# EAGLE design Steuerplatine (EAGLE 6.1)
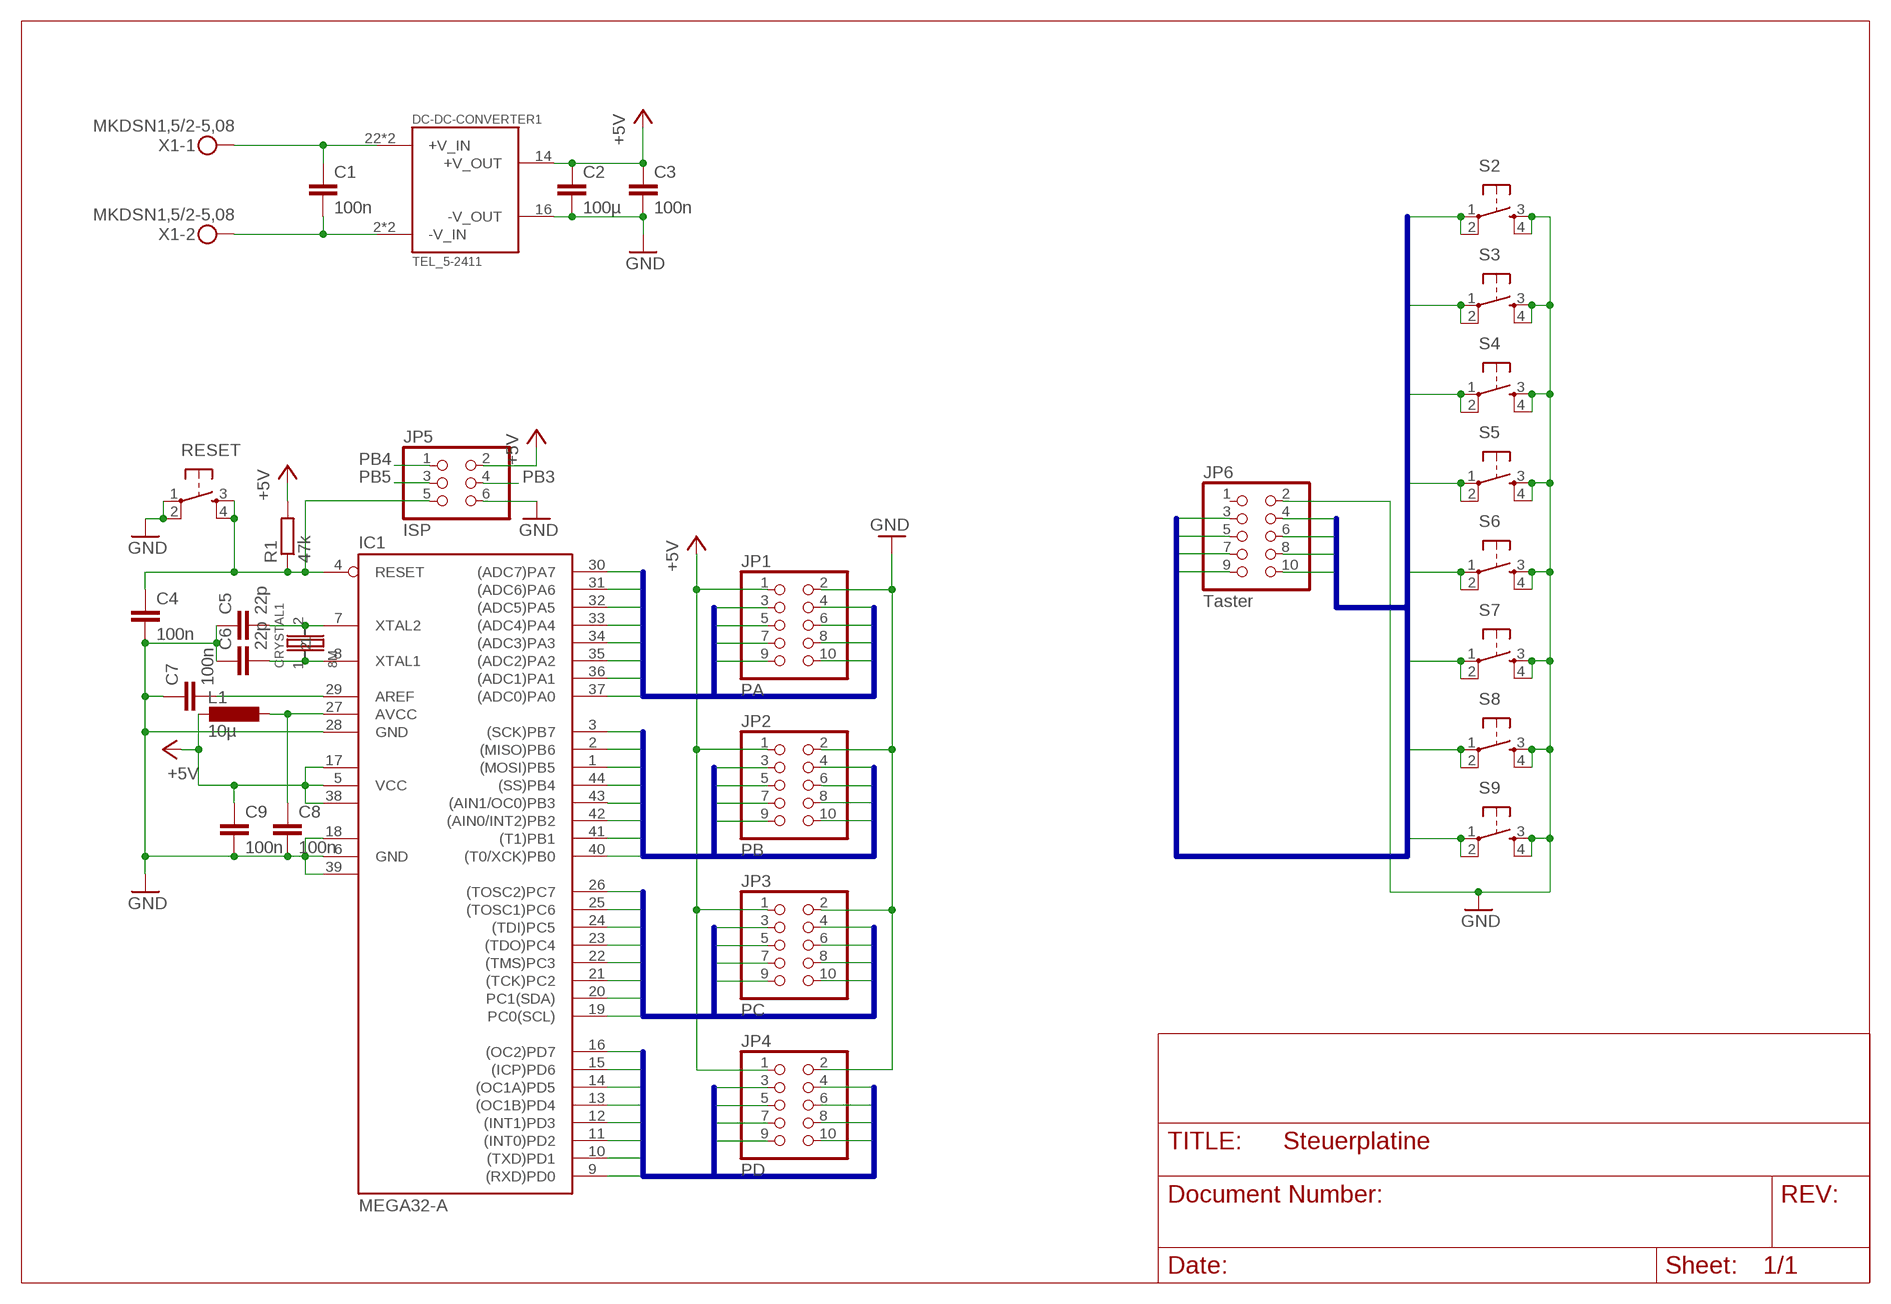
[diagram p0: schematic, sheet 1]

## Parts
C1  100n  C-EUC0603  [C0603]
C2  100µ  C-EUC1210  [C1210]
C3  100n  C-EUC0603  [C0603]
C4  100n  C-EUC0603  [C0603]
C5  22p  C-EUC0402  [C0402]
C6  22p  C-EUC0402  [C0402]
C7  100n  C-EUC0603  [C0603]
C8  100n  C-EUC0603  [C0603]
C9  100n  C-EUC0603  [C0603]
CRYSTAL1  8M  HC-49/SM  [HC-49/SM]
DC-DC-CONVERTER1  TEL_5-2411  [TEL_5-2411]
IC1  MEGA32-A  [TQFP44]
JP1  PA  PINHD-2X5  [2X05]
JP2  PB  PINHD-2X5  [2X05]
JP3  PC  PINHD-2X5  [2X05]
JP4  PD  PINHD-2X5  [2X05]
JP5  ISP  PINHD-2X3  [2X03]
JP6  Taster  PINHD-2X5  [2X05]
L1  10µ  L-EUL1812  [L1812]
R1  47k  R-EU_R0402  [R0402]
RESET  LSG  [SCHURTER_LSG]
S2  LSG  [SCHURTER_LSG]
S3  LSG  [SCHURTER_LSG]
S4  LSG  [SCHURTER_LSG]
S5  LSG  [SCHURTER_LSG]
S6  LSG  [SCHURTER_LSG]
S7  LSG  [SCHURTER_LSG]
S8  LSG  [SCHURTER_LSG]
S9  LSG  [SCHURTER_LSG]
X1  MKDSN1,5/2-5,08  [MKDSN1,5/2-5,08]

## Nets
+5V [5V]: C2.1 C3.1 C9.1 DC-DC-CONVERTER1.14(+V_OUT) IC1.5(VCC) IC1.17(VCC1) IC1.38(VCC2) JP1.1 JP2.1 JP3.1 JP4.1 JP5.2 L1.2 R1.2
GND [5V]: C2.2 C3.2 C4.2 C5.1 C6.1 C7.1 C8.2 C9.2 DC-DC-CONVERTER1.16(-V_OUT) IC1.6(GND) IC1.18(GND1) IC1.28(GND) IC1.39(GND2) JP1.2 JP2.2 JP3.2 JP4.2 JP5.6 JP6.2 RESET.1(P) RESET.2(P1) S2.3(S) S2.4(S1) S3.3(S) S3.4(S1) S4.3(S) S4.4(S1) S5.3(S) S5.4(S1) S6.3(S) S6.4(S1) S7.3(S) S7.4(S1) S8.3(S) S8.4(S1) S9.3(S) S9.4(S1)
N$1 [24V In]: C1.1 DC-DC-CONVERTER1.22(+V_IN) DC-DC-CONVERTER1.23(+V_IN) X1.1
N$2 [24V In]: C1.2 DC-DC-CONVERTER1.2(-V_IN) DC-DC-CONVERTER1.3(-V_IN) X1.2
N$3 [5V]: C4.1 IC1.4(RESET) JP5.5 R1.1 RESET.3(S) RESET.4(S1)
N$4 [5V]: C5.2 CRYSTAL1.2 IC1.7(XTAL2)
N$5 [5V]: C6.2 CRYSTAL1.1 IC1.8(XTAL1)
N$6 [5V]: C7.2 IC1.29(AREF)
N$7: C8.1 IC1.27(AVCC) L1.1
PA0 [5V]: IC1.37((ADC0)PA0) JP1.3
PA1 [5V]: IC1.36((ADC1)PA1) JP1.4
PA2 [5V]: IC1.35((ADC2)PA2) JP1.5
PA3 [5V]: IC1.34((ADC3)PA3) JP1.6
PA4 [5V]: IC1.33((ADC4)PA4) JP1.7
PA5 [5V]: IC1.32((ADC5)PA5) JP1.8
PA6 [5V]: IC1.31((ADC6)PA6) JP1.9
PA7 [5V]: IC1.30((ADC7)PA7) JP1.10
PB0 [5V]: IC1.40((T0/XCK)PB0) JP2.3
PB1 [5V]: IC1.41((T1)PB1) JP2.4
PB2 [5V]: IC1.42((AIN0/INT2)PB2) JP2.5
PB3: IC1.43((AIN1/OC0)PB3) JP2.6 JP5.4
PB4: IC1.44((SS)PB4) JP2.7 JP5.1
PB5 [5V]: IC1.1((MOSI)PB5) JP2.8 JP5.3
PB6 [5V]: IC1.2((MISO)PB6) JP2.9
PB7 [5V]: IC1.3((SCK)PB7) JP2.10
PC0 [5V]: IC1.19(PC0(SCL)) JP3.3
PC1 [5V]: IC1.20(PC1(SDA)) JP3.4
PC2 [5V]: IC1.21((TCK)PC2) JP3.5
PC3 [5V]: IC1.22((TMS)PC3) JP3.6
PC4 [5V]: IC1.23((TDO)PC4) JP3.7
PC5 [5V]: IC1.24((TDI)PC5) JP3.8
PC6 [5V]: IC1.25((TOSC1)PC6) JP3.9
PC7 [5V]: IC1.26((TOSC2)PC7) JP3.10
PD0 [5V]: IC1.9((RXD)PD0) JP4.3
PD1 [5V]: IC1.10((TXD)PD1) JP4.4
PD2 [5V]: IC1.11((INT0)PD2) JP4.5
PD3 [5V]: IC1.12((INT1)PD3) JP4.6
PD4 [5V]: IC1.13((OC1B)PD4) JP4.7
PD5 [5V]: IC1.14((OC1A)PD5) JP4.8
PD6 [5V]: IC1.15((ICP)PD6) JP4.9
PD7 [5V]: IC1.16((OC2)PD7) JP4.10
TASTER3 [5V]: JP6.3 S2.1(P) S2.2(P1)
TASTER4 [5V]: JP6.4 S3.1(P) S3.2(P1)
TASTER5 [5V]: JP6.5 S4.1(P) S4.2(P1)
TASTER6 [5V]: JP6.6 S5.1(P) S5.2(P1)
TASTER7 [5V]: JP6.7 S6.1(P) S6.2(P1)
TASTER8 [5V]: JP6.8 S7.1(P) S7.2(P1)
TASTER9 [5V]: JP6.9 S8.1(P) S8.2(P1)
TASTER10 [5V]: JP6.10 S9.1(P) S9.2(P1)
Unconnected: JP6.1

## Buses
PA[0..7]
PB[0..7]
PC[0..7]
PD[0..7]
TASTER[1..10]

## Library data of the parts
C1-C9 = rcl:C-EU: CAPACITOR, European symbol
CRYSTAL1 = Bachelorarbeit_lib_Jonas:HC-49/SM: Quarz
DC-DC-CONVERTER1 = Bachelorarbeit_lib_Jonas:TEL_5-2411: DCDC Wandler TRACOPOWER TEL 5-2411 Link http://de.farnell.com/tracopower/tel-5-2411/wandler-dc-dc-5w-5v/dp/1242622?Ntt=tel5+2411
IC1 = atmel:MEGA32: MICROCONTROLLER 32 Kbytes FLASH 2 Kbytes SRAM 1 Kbytes EEPROM USART 8-channel 10 bit ADC Source: www.atmel.com .. doc2503.pdf; MPN: ATMEGA32-16AU; OC_FARNELL: 9171274; OC_NEWARK: 69K6677
JP1-JP4 JP6 = pinhead:PINHD-2X5: PIN HEADER
JP5 = pinhead:PINHD-2X3: PIN HEADER
L1 = rcl:L-EU: INDUCTOR, European symbol
R1 = rcl:R-EU_: RESISTOR, European symbol
RESET S2-S9 = switch-omron-smd:LSG
X1 = con-phoenix-508:MKDSN1,5/2-5,08: MKDSN 1,5/ 2-5,08 Printklemme; MPN: MKDSN 1,5/2-5.08; OC_FARNELL: 1792903; OC_NEWARK: 30M2397

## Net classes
1 24V In: width 0.254 mm, drill 0.584 mm
2 5V: width 0.203 mm, drill 0.584 mm

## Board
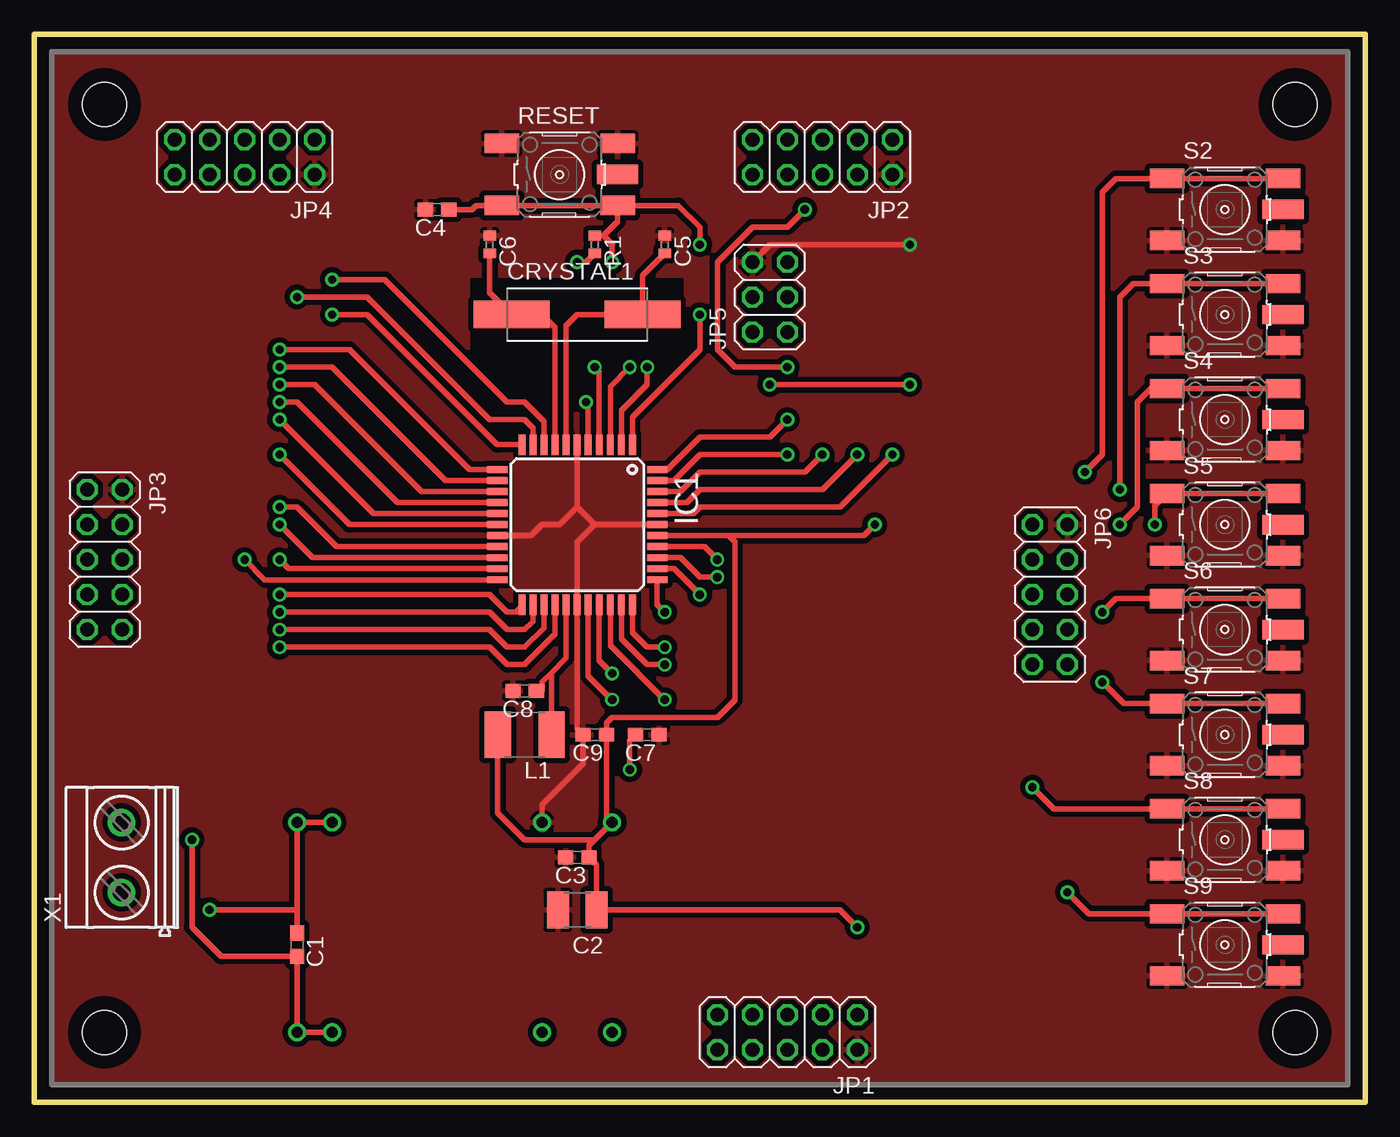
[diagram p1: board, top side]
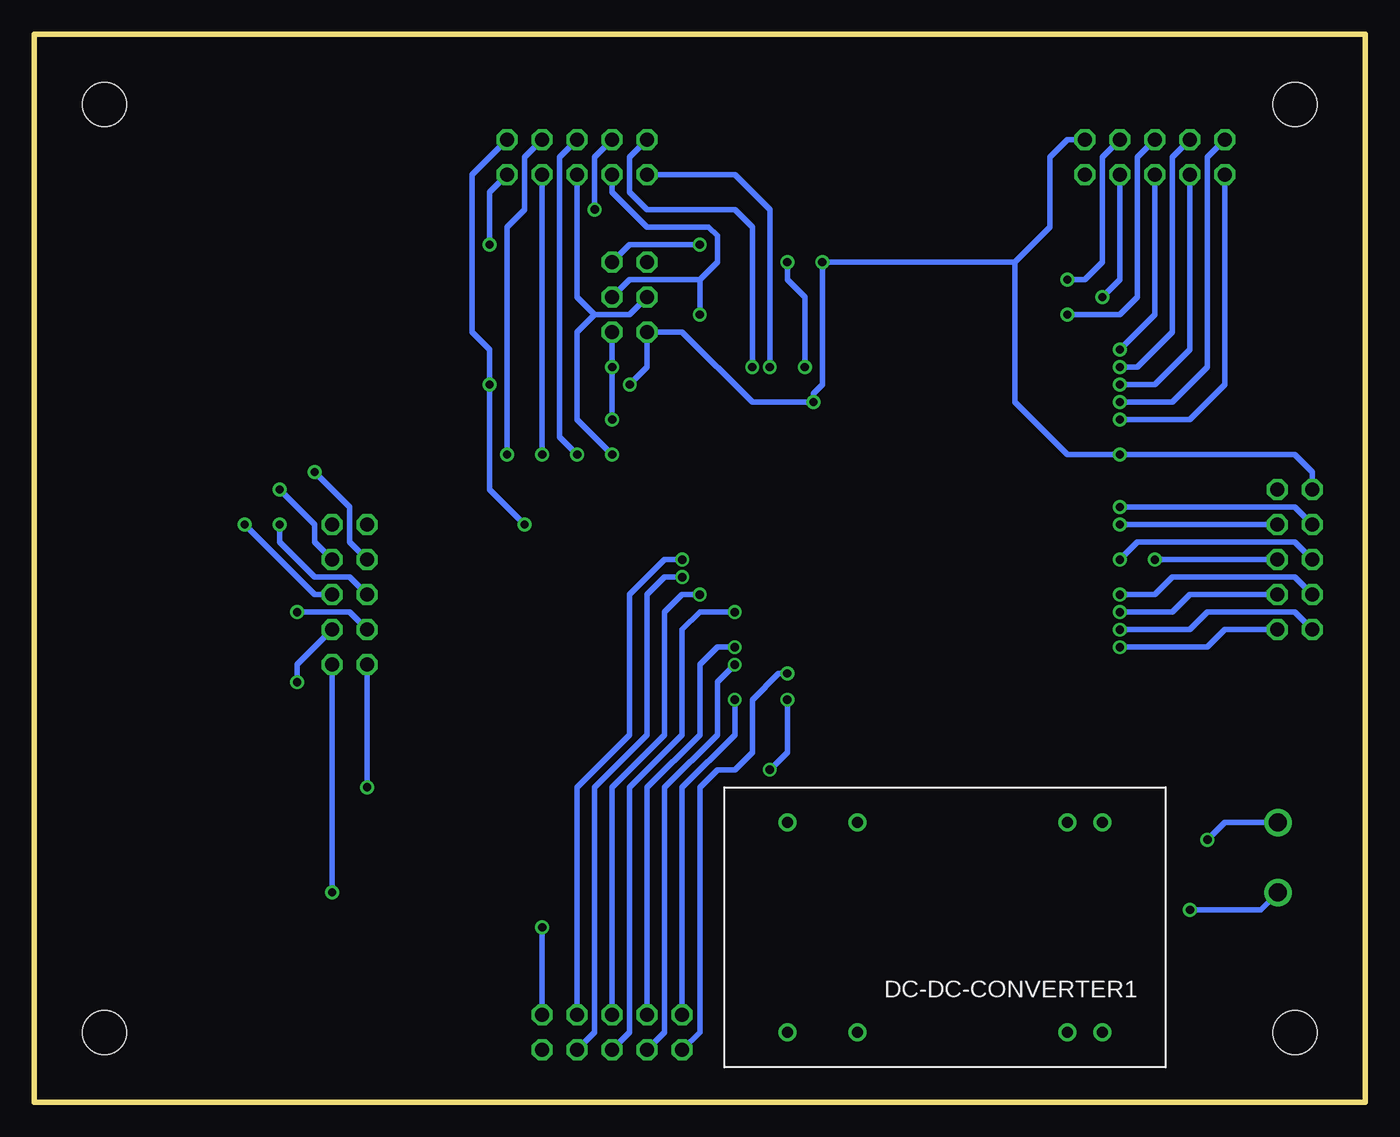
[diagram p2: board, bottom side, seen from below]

Size 96.52 x 77.47 mm. Coordinates in mm from the lower left corner, seen from the top.
Outline: 0,0 0,77.47 96.52,77.47 96.52,0 0,0
Copper layers (1*16): Top 0.035mm / dielectric 1.5mm / Bottom 0.035mm
Design rules: minimum track width 10mil, minimum drill 23mil, track to track 15mil, track to pad 12mil, pad to pad 8mil, via to via 8mil, smd to smd 8mil, copper to edge 40mil, drill to drill 8mil, minimum pad ring 10mil, minimum via ring 8mil, stop-mask expansion 4mil, vias tented up to drill 0mil, thermal gap 10mil
Holes 3.2 mm at 5.08,5.08 5.08,72.39 91.44,72.39 91.44,5.08
tRestrict: 4 lines

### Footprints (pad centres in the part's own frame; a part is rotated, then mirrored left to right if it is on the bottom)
C0603 = smd 1.1 x 1: 1 -0.85,0; 2 0.85,0
C1210 = smd 1.6 x 2.7: 1 -1.4,0; 2 1.4,0
C0402 = smd 0.7 x 0.9: 1 -0.65,0; 2 0.65,0
HC-49/SM = smd 5.499 x 2: 1 -4.75,0; 2 4.75,0
TEL_5-2411 = drill 0.8: 2 -11.43,7.62; 3 -8.89,7.62; 9 6.35,7.62; 11 11.43,7.62; 14 11.43,-7.62; 16 6.35,-7.62; 22 -8.89,-7.62; 23 -11.43,-7.62
TQFP44 = smd 1.5 x 0.5: 1 -5.8,4; 2 -5.8,3.2; 3 -5.8,2.4; 4 -5.8,1.6; 5 -5.8,0.8; 6 -5.8,0; 7 -5.8,-0.8; 8 -5.8,-1.6; 9 -5.8,-2.4; 10 -5.8,-3.2; 11 -5.8,-4; 23 5.8,-4; 24 5.8,-3.2; 25 5.8,-2.4; 26 5.8,-1.6; 27 5.8,-0.8; 28 5.8,0; 29 5.8,0.8; 30 5.8,1.6; 31 5.8,2.4; 32 5.8,3.2; 33 5.8,4 | smd 0.5 x 1.5: 12 -4,-5.8; 13 -3.2,-5.8; 14 -2.4,-5.8; 15 -1.6,-5.8; 16 -0.8,-5.8; 17 0,-5.8; 18 0.8,-5.8; 19 1.6,-5.8; 20 2.4,-5.8; 21 3.2,-5.8; 22 4,-5.8; 34 4,5.8; 35 3.2,5.8; 36 2.4,5.8; 37 1.6,5.8; 38 0.8,5.8; 39 0,5.8; 40 -0.8,5.8; 41 -1.6,5.8; 42 -2.4,5.8; 43 -3.2,5.8; 44 -4,5.8
2X05 = drill 1.016 octagon: 1 -5.08,-1.27; 2 -5.08,1.27; 3 -2.54,-1.27; 4 -2.54,1.27; 5 0,-1.27; 6 0,1.27; 7 2.54,-1.27; 8 2.54,1.27; 9 5.08,-1.27; 10 5.08,1.27
2X03 = drill 1.016 octagon: 1 -2.54,-1.27; 2 -2.54,1.27; 3 0,-1.27; 4 0,1.27; 5 2.54,-1.27; 6 2.54,1.27
L1812 = smd 1.9 x 3.4: 1 -1.95,0; 2 1.95,0
R0402 = smd 0.7 x 0.9: 1 -0.65,0; 2 0.65,0
SCHURTER_LSG = smd 2.5 x 1.4: 1 -4.2,2.25; 2 4.2,2.25; 3 -4.2,-2.25; 4 4.2,-2.25 | smd 3 x 1.4: 5 4.2,0
MKDSN1,5/2-5,08 = drill 1.3 pad 2: 1 -2.561,0.025; 2 2.519,0.025

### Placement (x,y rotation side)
C1  19.05,11.43 270 top
C2  39.37,13.97 180 top
C3  39.37,17.78 180 top
C4  29.21,64.77 180 top
C5  45.72,62.23 270 top
C6  33.02,62.23 270 top
C7  44.45,26.67 180 top
C8  35.56,29.84 180 top
C9  40.64,26.67 180 top
CRYSTAL1  39.37,57.15 0 top
DC-DC-CONVERTER1  30.48,12.7 180 bottom
IC1  39.37,41.91 270 top
JP1  54.61,5.08 180 top
JP2  57.15,68.58 180 top
JP3  5.08,39.37 270 top
JP4  15.24,68.58 180 top
JP5  53.34,58.42 90 top
JP6  73.66,36.83 270 top
L1  35.56,26.67 180 top
R1  40.64,62.23 270 top
RESET  38.1,67.31 0 top
S2  86.36,64.77 0 top
S3  86.36,57.15 0 top
S4  86.36,49.53 0 top
S5  86.36,41.91 0 top
S6  86.36,34.29 0 top
S7  86.36,26.67 0 top
S8  86.36,19.05 0 top
S9  86.36,11.43 0 top
X1  6.35,17.78 90 top

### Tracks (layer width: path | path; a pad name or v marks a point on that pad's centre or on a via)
+5V  (via drill 0.6)
  Top 0.406: 40.64,19.05 40.22,18.63 C3.1 40.77,17.23 C2.1 58.42,13.97 v59.69,12.7 | L1.2 33.61,21 35.56,19.05 40.64,19.05 | 40.64,19.05 DC-DC-CONVERTER1.14 41.49,20.74 C9.1 41.49,27.52 41.91,27.94 49.53,27.94 50.8,29.21 50.8,40.64 50.33,41.11 IC1.38 60.16,41.11 v60.96,41.91 | IC1.5 40.17,50.64 v40.01,50.8 | v39.37,60.96 40.02,60.96 R1.2 | IC1.17 22.86,41.91 v17.78,46.99 | v53.34,52.07 v63.5,52.07
  Bottom 0.406: JP2.1 64.77,67.31 64.77,55.88 63.5,54.61 v63.5,52.07 63.5,44.45 v60.96,41.91 | JP1.1 v59.69,12.7 | 25.4,60.96 v39.37,60.96 39.37,52.07 40.01,51.44 v40.01,50.8 44.45,50.8 49.53,55.88 JP5.2 52.07,53.34 v53.34,52.07 | 25.4,60.96 22.86,63.5 22.86,68.58 21.59,69.85 JP4.1 | JP3.1 3.81,45.72 5.08,46.99 v17.78,46.99 21.59,46.99 25.4,50.8 25.4,60.96
GND  (via drill 0.6)
  Top 0.406: DC-DC-CONVERTER1.16 36.83,21.59 39.79,24.55 C9.2 39.37,27.09 IC1.28 39.37,40.64 40.64,41.91 | IC1.39 40.64,41.91 | 40.64,41.91 39.37,43.18 | 39.37,43.18 IC1.6 | IC1.18 36.03,41.11 36.83,41.91 38.1,41.91 39.37,43.18 | JP5.6 53.34,62.23 v63.5,62.23
  Bottom 0.406: v63.5,62.23 63.5,66.04 JP2.2
  pour Top (rank 6): 95.25,76.2 1.27,76.2 1.27,1.27 95.25,1.27
N$1  (via drill 0.6)
  Top 0.406: C1.1 19.05,13.97 | 19.05,13.97 v12.7,13.97 | 19.05,13.97 DC-DC-CONVERTER1.23 DC-DC-CONVERTER1.22
  Bottom 0.406: v12.7,13.97 7.57,13.97 X1.1
N$2  (via drill 0.6)
  Top 0.406: v11.43,19.05 11.43,12.7 13.55,10.58 C1.2 DC-DC-CONVERTER1.2 DC-DC-CONVERTER1.3
  Bottom 0.406: X1.2 10.18,20.3 v11.43,19.05
N$3  (via drill 0.6)
  Top 0.406: RESET.4 RESET.3 32.04,65.06 31.75,64.77 C4.1 | R1.1 41.29,62.88 | 41.29,62.88 42.3,63.89 RESET.4 | IC1.4 40.97,53.01 v40.64,53.34 | v41.91,60.96 41.91,62.26 | 41.91,62.26 41.29,62.88 | 41.94,62.23 41.91,62.26 | v48.26,62.23 48.26,63.5 46.7,65.06 RESET.4
  Bottom 0.406: v40.64,53.34 40.64,58.42 41.91,59.69 v41.91,60.96 | JP5.5 53.34,62.23 v48.26,62.23
N$4
  Top 0.406: IC1.7 38.57,56.35 39.37,57.15 CRYSTAL1.2 44.12,59.98 C5.2
N$5
  Top 0.406: IC1.8 37.77,56.21 36.83,57.15 CRYSTAL1.1 33.02,58.75 C6.2
N$6  (via drill 0.6)
  Top 0.406: IC1.29 40.17,30.95 v41.91,29.21 | v43.18,24.13 43.18,26.25 C7.2
  Bottom 0.406: v41.91,29.21 41.91,25.4 v43.18,24.13
N$7
  Top 0.406: L1.1 37.51,31.16 | 37.51,31.16 38.57,32.22 IC1.27 | C8.1 36.83,29.84 36.83,30.48 37.51,31.16
PA0  (via drill 0.6)
  Top 0.406: IC1.37 48.59,40.31 v49.53,39.37
  Bottom 0.406: v49.53,39.37 50.8,39.37 53.34,36.83 53.34,26.67 57.15,22.86 JP1.3
PA1  (via drill 0.6)
  Top 0.406: IC1.36 46.85,39.51 48.26,38.1 v49.53,38.1
  Bottom 0.406: JP1.4 55.88,5.08 55.88,22.86 52.07,26.67 52.07,36.83 50.8,38.1 v49.53,38.1
PA2  (via drill 0.6)
  Top 0.406: IC1.35 46.38,38.71 v48.26,36.83
  Bottom 0.406: JP1.5 54.61,22.86 50.8,26.67 50.8,35.56 49.53,36.83 v48.26,36.83
PA3  (via drill 0.6)
  Top 0.406: IC1.34 45.17,36.11 v45.72,35.56
  Bottom 0.406: JP1.6 53.34,5.08 53.34,22.86 49.53,26.67 49.53,34.29 48.26,35.56 v45.72,35.56
PA4  (via drill 0.6)
  Top 0.406: IC1.33 43.37,34.1 44.45,33.02 v45.72,33.02
  Bottom 0.406: v45.72,33.02 46.99,33.02 48.26,31.75 48.26,26.67 52.07,22.86 JP1.7
PA5  (via drill 0.6)
  Top 0.406: IC1.32 42.57,33.63 44.45,31.75 v45.72,31.75
  Bottom 0.406: v45.72,31.75 46.99,30.48 46.99,26.67 50.8,22.86 50.8,5.08 JP1.8
PA6  (via drill 0.6)
  Top 0.406: v45.72,29.21 41.77,33.16 IC1.31
  Bottom 0.406: v45.72,29.21 45.72,26.67 49.53,22.86 JP1.9
PA7  (via drill 0.6)
  Top 0.406: IC1.30 40.97,32.05 v41.91,31.11
  Bottom 0.406: JP1.10 48.26,5.08 48.26,22.86 46.99,24.13 45.72,24.13 44.45,25.4 44.45,29.21 42.55,31.11 v41.91,31.11
PB0  (via drill 0.6)
  Top 0.406: IC1.40 47.79,42.71 48.26,43.18 58.42,43.18 v62.23,46.99
  Bottom 0.406: v62.23,46.99 62.23,63.5 60.96,64.77 60.96,68.58 JP2.3
PB1  (via drill 0.6)
  Top 0.406: IC1.41 47.32,43.51 48.26,44.45 57.15,44.45 v59.69,46.99
  Bottom 0.406: v59.69,46.99 JP2.4
PB2  (via drill 0.6)
  Top 0.406: IC1.42 46.85,44.31 48.26,45.72 55.88,45.72 v57.15,46.99
  Bottom 0.406: v57.15,46.99 58.42,48.26 58.42,68.58 JP2.5
PB3  (via drill 0.6)
  Top 0.406: IC1.43 46.38,45.11 48.26,46.99 v54.61,46.99
  Bottom 0.406: v54.61,46.99 57.15,49.53 57.15,55.88 55.88,57.15 | 55.88,57.15 53.34,57.15 JP5.4 | JP2.6 57.15,58.42 55.88,57.15
PB4  (via drill 0.6)
  Top 0.406: IC1.44 45.91,45.91 48.26,48.26 53.34,48.26 v54.61,49.53 | v55.88,64.77 54.61,63.5 52.07,63.5 49.53,60.96 49.53,54.61 50.8,53.34 v54.61,53.34
  Bottom 0.406: v54.61,49.53 v54.61,53.34 JP5.1 | JP2.7 55.88,68.58 v55.88,64.77
PB5  (via drill 0.6)
  Top 0.406: IC1.1 43.37,49.72 48.26,54.61 v48.26,57.15
  Bottom 0.406: JP5.3 53.34,59.69 48.26,59.69 | JP2.8 54.61,66.04 52.07,63.5 47.62,63.5 46.99,62.87 46.99,60.96 48.26,59.69 | v48.26,57.15 48.26,59.69
PB6  (via drill 0.6)
  Top 0.406: IC1.2 42.57,50.19 44.45,52.07 v44.45,53.34
  Bottom 0.406: v44.45,53.34 44.45,63.5 45.72,64.77 52.07,64.77 53.34,66.04 53.34,68.58 JP2.9
PB7  (via drill 0.6)
  Top 0.406: IC1.3 41.77,51.93 v43.18,53.34
  Bottom 0.406: v43.18,53.34 43.18,64.77 45.72,67.31 JP2.10
PC0  (via drill 0.6)
  Top 0.406: IC1.19 21.92,40.31 19.05,43.18 v17.78,43.18
  Bottom 0.406: v17.78,43.18 5.08,43.18 JP3.3
PC1  (via drill 0.6)
  Top 0.406: IC1.20 20.18,39.51 v17.78,41.91
  Bottom 0.406: JP3.4 v17.78,41.91
PC2  (via drill 0.6)
  Top 0.406: IC1.21 18.44,38.71 v17.78,39.37
  Bottom 0.406: v17.78,39.37 16.51,40.64 5.08,40.64 JP3.5
PC3  (via drill 0.6)
  Top 0.406: IC1.22 16.7,37.91 v15.24,39.37
  Bottom 0.406: v15.24,39.37 JP3.6
PC4  (via drill 0.6)
  Top 0.406: v17.78,36.83 33.02,36.83 34.29,35.56 34.93,35.56 35.37,36.01 IC1.23
  Bottom 0.406: JP3.7 5.08,38.1 13.97,38.1 15.24,36.83 v17.78,36.83
PC5  (via drill 0.6)
  Top 0.406: v17.78,35.56 33.02,35.56 34.29,34.29 35.56,34.29 36.17,34.9 IC1.24
  Bottom 0.406: JP3.8 12.7,36.83 13.97,35.56 v17.78,35.56
PC6  (via drill 0.6)
  Top 0.406: v17.78,34.29 33.02,34.29 34.29,33.02 35.56,33.02 36.97,34.43 IC1.25
  Bottom 0.406: JP3.9 5.08,35.56 11.43,35.56 12.7,34.29 v17.78,34.29
PC7  (via drill 0.6)
  Top 0.406: v17.78,33.02 33.02,33.02 34.29,31.75 35.56,31.75 37.77,33.96 IC1.26
  Bottom 0.406: JP3.10 10.16,34.29 11.43,33.02 v17.78,33.02
PD0  (via drill 0.6)
  Top 0.406: IC1.9 36.97,49.39 35.56,50.8 34.29,50.8 25.4,59.69 v21.59,59.69
  Bottom 0.406: v21.59,59.69 20.32,59.69 19.05,60.96 19.05,68.58 JP4.3
PD1  (via drill 0.6)
  Top 0.406: IC1.10 36.17,48.92 35.56,49.53 33.02,49.53 24.13,58.42 v19.05,58.42
  Bottom 0.406: v19.05,58.42 17.78,59.69 JP4.4
PD2  (via drill 0.6)
  Top 0.406: IC1.11 33.57,47.71 24.13,57.15 v21.59,57.15
  Bottom 0.406: JP4.5 16.51,68.58 16.51,58.42 17.78,57.15 v21.59,57.15
PD3  (via drill 0.6)
  Top 0.406: IC1.12 31.56,45.91 22.86,54.61 v17.78,54.61
  Bottom 0.406: JP4.6 15.24,57.15 v17.78,54.61
PD4  (via drill 0.6)
  Top 0.406: IC1.13 29.82,45.11 21.59,53.34 v17.78,53.34
  Bottom 0.406: v17.78,53.34 16.51,53.34 13.97,55.88 13.97,68.58 JP4.7
PD5  (via drill 0.6)
  Top 0.406: IC1.14 28.08,44.31 20.32,52.07 v17.78,52.07
  Bottom 0.406: v17.78,52.07 15.24,52.07 12.7,54.61 JP4.8
PD6  (via drill 0.6)
  Top 0.406: IC1.15 26.34,43.51 19.05,50.8 v17.78,50.8
  Bottom 0.406: v17.78,50.8 13.97,50.8 11.43,53.34 11.43,68.58 JP4.9
PD7  (via drill 0.6)
  Top 0.406: IC1.16 24.6,42.71 v17.78,49.53
  Bottom 0.406: v17.78,49.53 12.7,49.53 10.16,52.07 JP4.10
TASTER3  (via drill 0.6)
  Top 0.406: S2.2 S2.1 78.45,67.02 77.47,66.04 77.47,46.99 v76.2,45.72
  Bottom 0.406: v76.2,45.72 73.66,43.18 73.66,40.64 JP6.3
TASTER4  (via drill 0.6)
  Top 0.406: S3.2 S3.1 79.72,59.4 78.74,58.42 v78.74,44.45
  Bottom 0.406: v78.74,44.45 76.2,41.91 76.2,40.64 JP6.4
TASTER5  (via drill 0.6)
  Top 0.406: S4.2 S4.1 80.99,51.78 80.01,50.8 80.01,43.18 v78.74,41.91
  Bottom 0.406: v78.74,41.91 78.74,40.64 76.2,38.1 73.66,38.1 JP6.5
TASTER6  (via drill 0.6)
  Top 0.406: S5.2 S5.1 81.28,43.28 v81.28,41.91
  Bottom 0.406: JP6.6 76.2,36.83 v81.28,41.91
TASTER7  (via drill 0.6)
  Top 0.406: v77.47,35.56 78.45,36.54 S6.1 82.26,36.54 82.55,36.83 82.55,36.2 82.89,36.54 S6.2
  Bottom 0.406: v77.47,35.56 73.66,35.56 JP6.7
TASTER8  (via drill 0.6)
  Top 0.406: S7.2 S7.1 79.03,28.92 v77.47,30.48
  Bottom 0.406: v77.47,30.48 77.47,31.75 JP6.8
TASTER9  (via drill 0.6)
  Top 0.406: S8.2 S8.1 73.95,21.3 v72.39,22.86
  Bottom 0.406: v72.39,22.86 JP6.9
TASTER10  (via drill 0.6)
  Top 0.406: S9.2 S9.1 76.49,13.68 v74.93,15.24
  Bottom 0.406: v74.93,15.24 JP6.10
